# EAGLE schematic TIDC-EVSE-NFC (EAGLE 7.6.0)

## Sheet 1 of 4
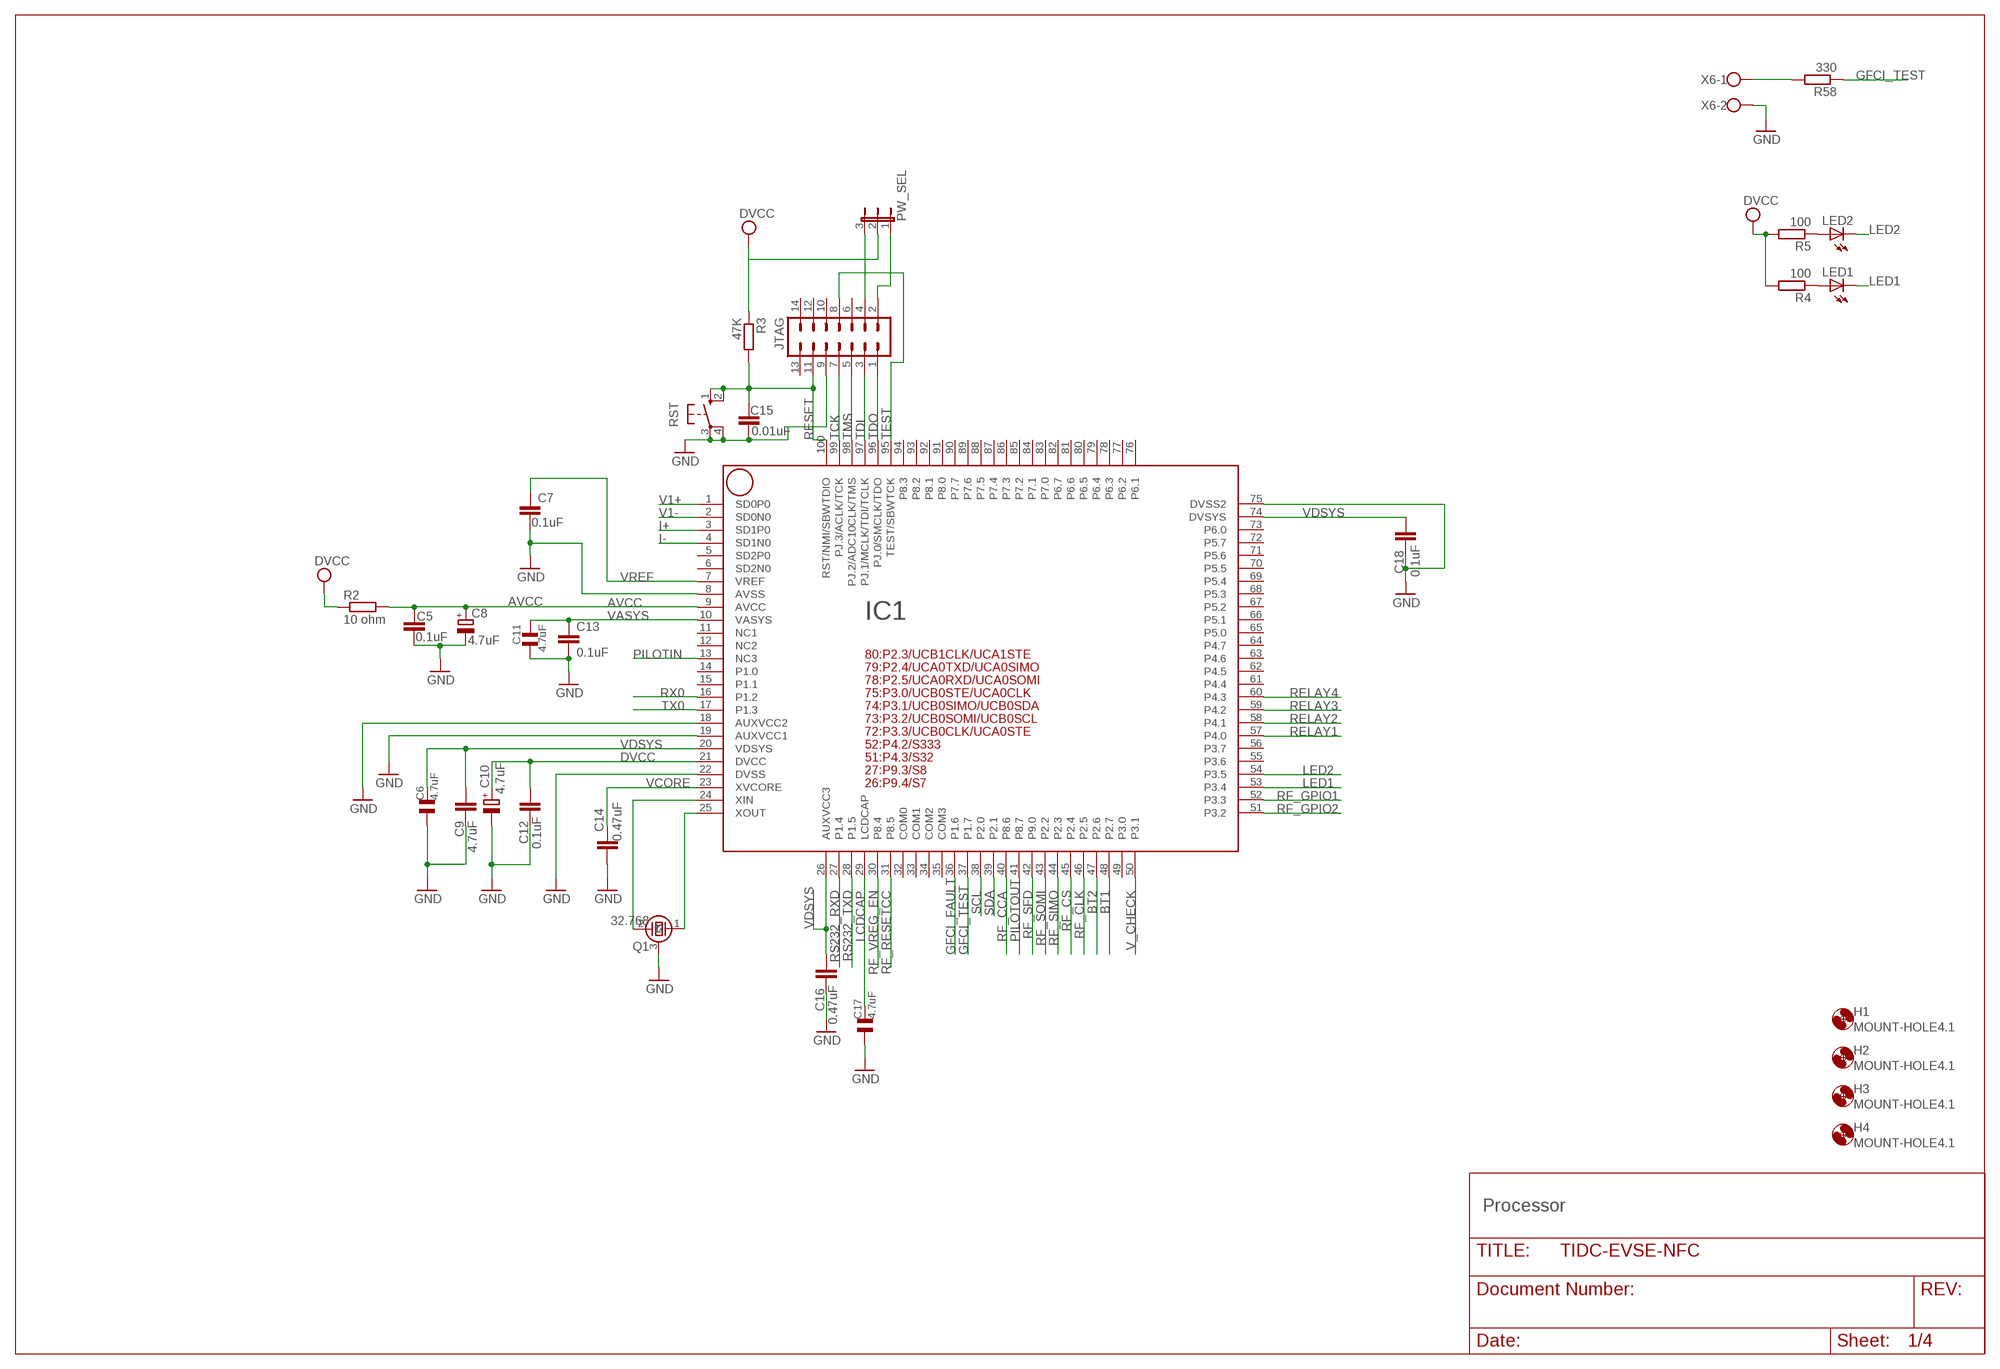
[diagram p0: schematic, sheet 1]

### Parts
C5  0.1uF  C-EUC0603  [C0603]
C6  4.7uF  C_0805  [0805]
C7  0.1uF  C-EUC0603  [C0603]
C8  4.7uF  CPOL-EUSMCB  [SMC_B]
C9  4.7uF  C-EUC0603  [C0603]
C10  4.7uF  CPOL-EUSMCB  [SMC_B]
C11  4.7uF  C_0805  [0805]
C12  0.1uF  C-EUC0603  [C0603]
C13  0.1uF  C-EUC0603  [C0603]
C14  0.47uF  C-EUC0603  [C0603]
C15  0.01uF  C-EUC0603  [C0603]
C16  0.47uF  C-EUC0603  [C0603]
C17  4.7uF  C_0805  [0805]
C18  0.1uF  C-EUC0603  [C0603]
H1  MOUNT-HOLE4.1  [4,1]
H2  MOUNT-HOLE4.1  [4,1]
H3  MOUNT-HOLE4.1  [4,1]
H4  MOUNT-HOLE4.1  [4,1]
IC1  F6733---PZ100  [PZ100]
JTAG  MA07-2MA07-2JTAG  [MA07-2JTAG]
LED1  LED3MM  [LED3MM]
LED2  LED3MM  [LED3MM]
PW_SEL  JP2E  [JP2]
Q1  32.768  CRYSTAL-LSDTC26H-1  [TC26H-1]
R2  10 ohm  R-EU_R0603  [R0603]
R3  47K  R-EU_R0603  [R0603]
R4  100  R-EU_R0603  [R0603]
R5  100  R-EU_R0603  [R0603]
R58  330  R-EU_R0603  [R0603]
RST  10-XX  [B3F-10XX]
X6  W237-102  [W237-102]

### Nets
AVCC: C5.1 C8.+ IC1.9(AVCC) R2.2 ; also sheet 4
BT1: IC1.48(P2.7) ; also sheet 2
BT2: IC1.47(P2.6) ; also sheet 2
DVCC: C10.+ C12.2 IC1.21(DVCC) PW_SEL.2 R2.1 R3.1 R4.2 R5.2 ; also sheet 2,3,4
GFCI_FAULT: IC1.36(P1.6) ; also sheet 4
GFCI_TEST: IC1.37(P1.7) R58.1
GND: C5.2 C6.1 C7.2 C8.- C9.1 C10.- C11.1 C12.1 C13.2 C14.1 C15.2 C16.1 C17.1 C18.1 IC1.8(AVSS) IC1.18(AUXVCC2) IC1.19(AUXVCC1) IC1.22(DVSS) IC1.75(DVSS2) JTAG.9 Q1.3 RST.3(P) RST.4(P1) X6.2 ; also sheet 2,3,4
I+: IC1.3(SD1P0) ; also sheet 4
I-: IC1.4(SD1N0) ; also sheet 4
JTAG_EXT: JTAG.4 PW_SEL.3
JTAG_INT: JTAG.2 PW_SEL.1
LCDCAP: C17.2 IC1.29(LCDCAP)
LED1: IC1.53(P3.4) LED1.K(C)
LED2: IC1.54(P3.5) LED2.K(C)
N$6: R58.2 X6.1
N$104: LED1.A R4.1
N$105: LED2.A R5.1
PILOTIN: IC1.13(NC3) ; also sheet 2
PILOTOUT: IC1.41(P8.7) ; also sheet 2
RELAY1: IC1.57(P4.0) ; also sheet 4
RELAY2: IC1.58(P4.1) ; also sheet 4
RELAY3: IC1.59(P4.2) ; also sheet 4
RELAY4: IC1.60(P4.3) ; also sheet 4
RESET: C15.1 IC1.100(RST/NMI/SBWTDIO) JTAG.11 R3.2 RST.1(S) RST.2(S1)
RF_CCA: IC1.40(P8.6) ; also sheet 2
RF_CLK: IC1.46(P2.5) ; also sheet 2
RF_CS: IC1.45(P2.4) ; also sheet 2
RF_GPIO1: IC1.52(P3.3) ; also sheet 2
RF_GPIO2: IC1.51(P3.2) ; also sheet 2
RF_RESETCC: IC1.31(P8.5) ; also sheet 2
RF_SFD: IC1.42(P9.0) ; also sheet 2
RF_SIMO: IC1.44(P2.3) ; also sheet 2
RF_SOMI: IC1.43(P2.2) ; also sheet 2
RF_VREG_EN: IC1.30(P8.4) ; also sheet 2
RS232_RXD: IC1.27(P1.4)
RS232_TXD: IC1.28(P1.5)
RX0: IC1.16(P1.2) ; also sheet 2
SCL: IC1.38(P2.0) ; also sheet 2
SDA: IC1.39(P2.1) ; also sheet 2
TCK: IC1.99(PJ.3/ACLK/TCK) JTAG.7
TDI: IC1.97(PJ.1/MCLK/TDI/TCLK) JTAG.3
TDO: IC1.96(PJ.0/SMCLK/TDO) JTAG.1
TEST: IC1.95(TEST/SBWTCK) JTAG.8
TMS: IC1.98(PJ.2/ADC10CLK/TMS) JTAG.5
TX0: IC1.17(P1.3) ; also sheet 2
V1+: IC1.1(SD0P0) ; also sheet 4
V1-: IC1.2(SD0N0) ; also sheet 4
V_CHECK: IC1.50(P3.1) ; also sheet 4
VASYS: C11.2 C13.1 IC1.10(VASYS)
VCORE: C14.2 IC1.23(XVCORE)
VDSYS: C6.2 C9.2 C16.2 C18.2 IC1.20(VDSYS) IC1.26(AUXVCC3) IC1.74(DVSYS)
VREF: C7.1 IC1.7(VREF)
XIN1: IC1.24(XIN) Q1.2
XOUT1: IC1.25(XOUT) Q1.1
Unconnected: IC1.5(SD2P0) IC1.6(SD2N0) IC1.11(NC1) IC1.12(NC2) IC1.14(P1.0) IC1.15(P1.1) IC1.32(COM0) IC1.33(COM1) IC1.34(COM2) IC1.35(COM3) IC1.49(P3.0) IC1.55(P3.6) IC1.56(P3.7) IC1.61(P4.4) IC1.62(P4.5) IC1.63(P4.6) IC1.65(P5.0) IC1.66(P5.1) IC1.68(P5.3) IC1.69(P5.4) IC1.70(P5.5) IC1.71(P5.6) IC1.72(P5.7) IC1.73(P6.0) IC1.76(P6.1) IC1.77(P6.2) IC1.78(P6.3) IC1.79(P6.4) IC1.80(P6.5) IC1.81(P6.6) IC1.82(P6.7) IC1.83(P7.0) IC1.84(P7.1) IC1.85(P7.2) IC1.86(P7.3) IC1.87(P7.4) IC1.88(P7.5) IC1.89(P7.6) IC1.90(P7.7) IC1.91(P8.0) IC1.93(P8.2) IC1.94(P8.3) JTAG.6 JTAG.10 JTAG.12 JTAG.13 JTAG.14

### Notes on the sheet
- Processor

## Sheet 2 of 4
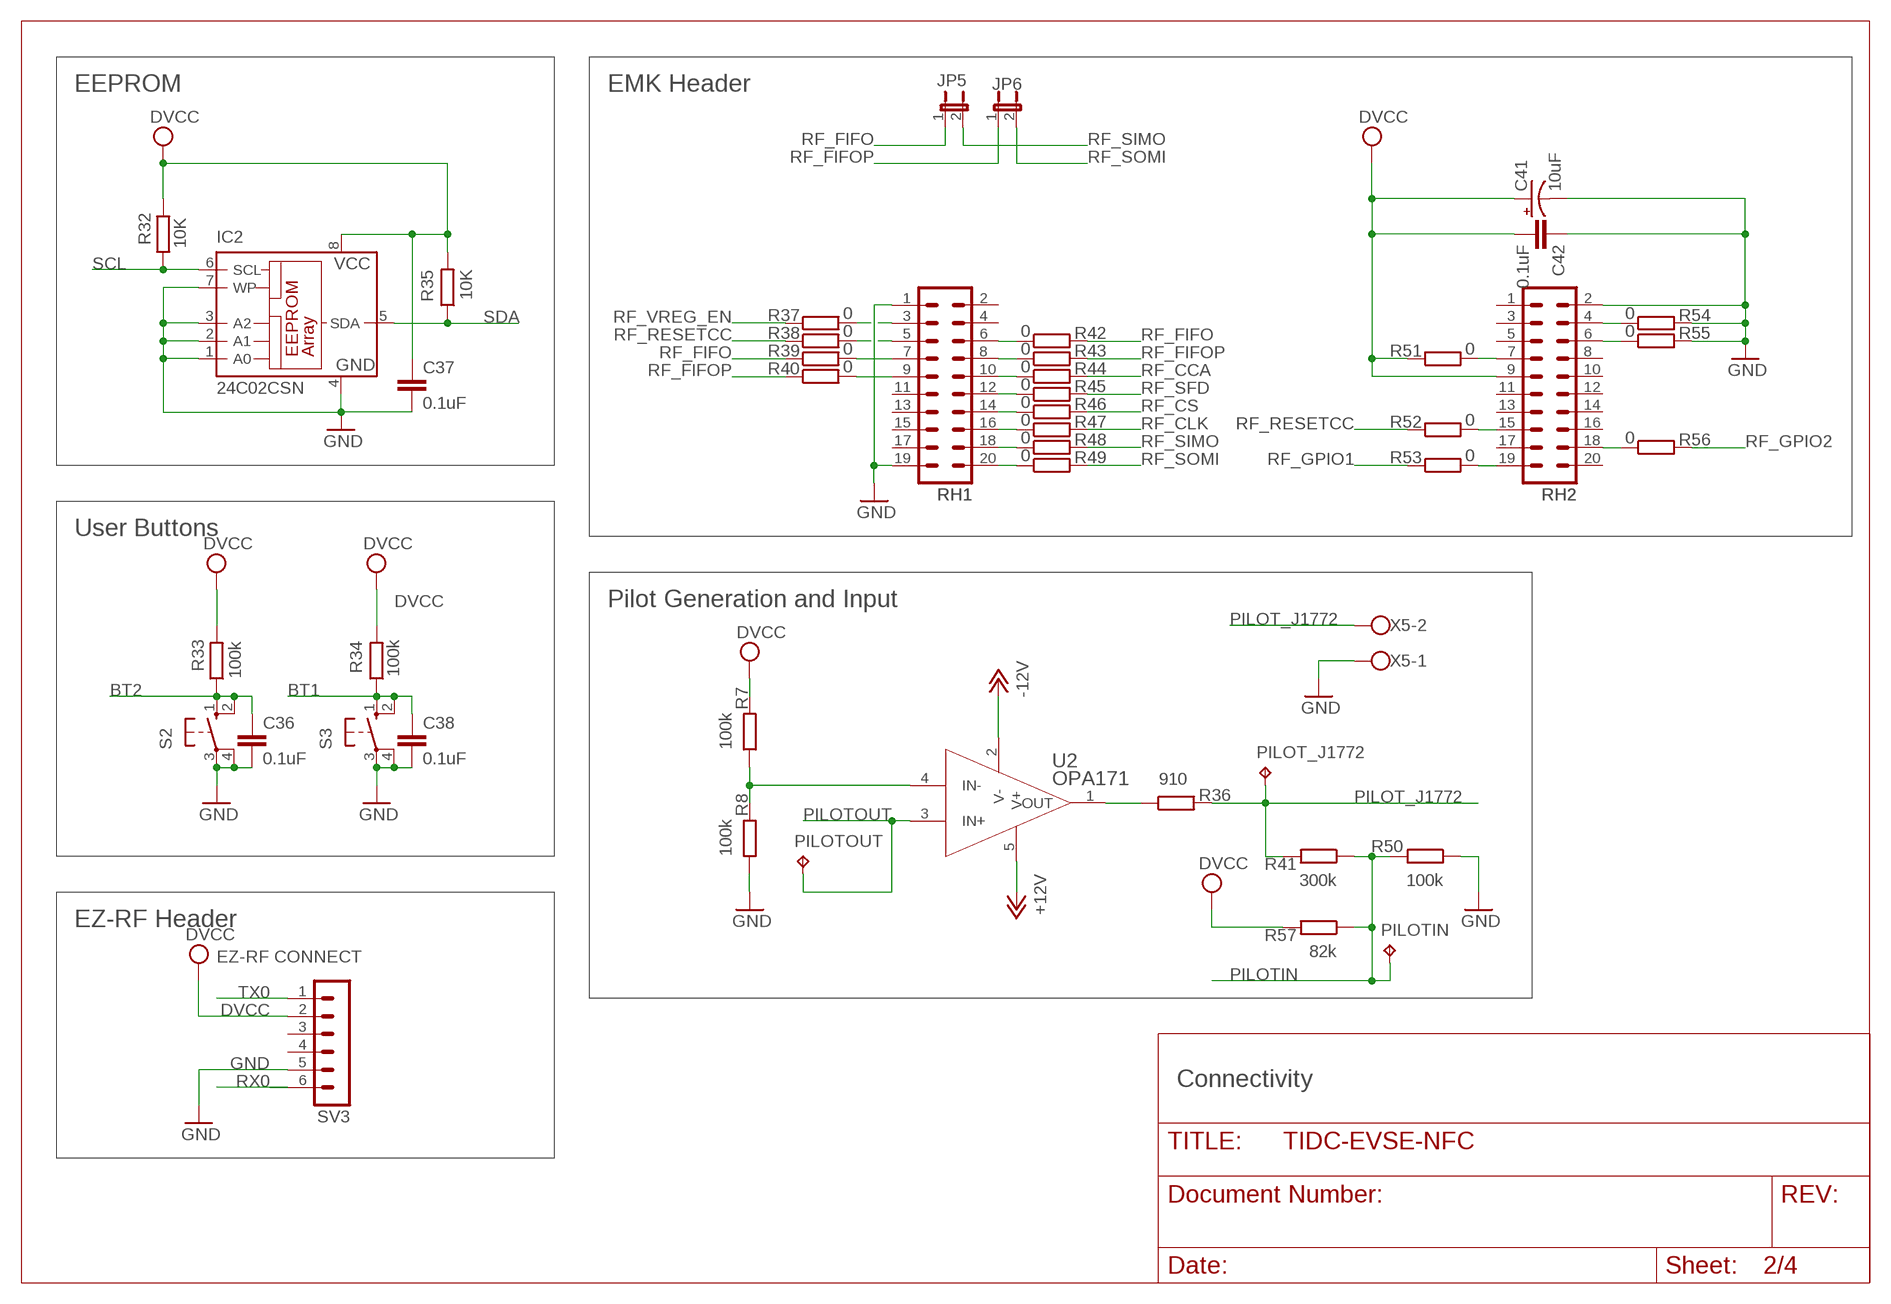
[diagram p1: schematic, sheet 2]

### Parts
C36  0.1uF  C-EUC0603  [C0603]
C37  0.1uF  C-EUC0603  [C0603]
C38  0.1uF  C-EUC0603  [C0603]
C41  10uF  CPOL-USCT3216  [CT3216]
C42  0.1uF  C-EUC0603  [C0603]
IC2  24C02CSN  [SO-08]
JP5  JP1E  [JP1]
JP6  JP1E  [JP1]
PILOT_J1772  TPB1,27  [B1,27]
PILOTIN  TPB1,27  [B1,27]
PILOTOUT  TPB1,27  [B1,27]
R7  100k  R-EU_R0603  [R0603]
R8  100k  R-EU_R0603  [R0603]
R32  10K  R-EU_R0603  [R0603]
R33  100k  R-EU_R0603  [R0603]
R34  100k  R-EU_R0603  [R0603]
R35  10K  R-EU_R0603  [R0603]
R36  910  R-EU_R0603  [R0603]
R37  0  R-EU_R0603  [R0603]
R38  0  R-EU_R0603  [R0603]
R39  0  R-EU_R0603  [R0603]
R40  0  R-EU_R0603  [R0603]
R41  300k  R-EU_R0603  [R0603]
R42  0  R-EU_R0603  [R0603]
R43  0  R-EU_R0603  [R0603]
R44  0  R-EU_R0603  [R0603]
R45  0  R-EU_R0603  [R0603]
R46  0  R-EU_R0603  [R0603]
R47  0  R-EU_R0603  [R0603]
R48  0  R-EU_R0603  [R0603]
R49  0  R-EU_R0603  [R0603]
R50  100k  R-EU_R0603  [R0603]
R51  0  R-EU_R0603  [R0603]
R52  0  R-EU_R0603  [R0603]
R53  0  R-EU_R0603  [R0603]
R54  0  R-EU_R0603  [R0603]
R55  0  R-EU_R0603  [R0603]
R56  0  R-EU_R0603  [R0603]
R57  82k  R-EU_R0603  [R0603]
RH1  TFM-110-02-SM-D-A-K  [TFM-110-02-SM-D-A-K]
RH2  TFM-110-02-SM-D-A-K  [TFM-110-02-SM-D-A-K]
S2  10-XX  [B3F-10XX]
S3  10-XX  [B3F-10XX]
SV3  MA06-1MA06-1-1.27  [MA06-1-1.27]
U2  OPA171  OPA171_DBV_5  [DBV5]
X5  W237-102  [W237-102]

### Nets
+12V: U2.5(V+) ; also sheet 3,4
-12V: U2.2(V-) ; also sheet 3
BT1: C38.1 R34.1 S3.1(S) S3.2(S1) ; also sheet 1
BT2: C36.1 R33.1 S2.1(S) S2.2(S1) ; also sheet 1
DVCC: C37.1 C41.+ C42.2 IC2.8(VCC) R7.2 R32.2 R33.2 R34.2 R35.2 R51.1 R57.2 RH2.9 SV3.2 ; also sheet 1,3,4
GND: C36.2 C37.2 C38.2 C41.- C42.1 IC2.1(A0) IC2.2(A1) IC2.3(A2) IC2.4(GND) IC2.7(WP) R8.1 R50.1 R54.2 R55.2 RH1.1 RH1.19 RH2.2 S2.3(P) S2.4(P1) S3.3(P) S3.4(P1) SV3.5 X5.1 ; also sheet 1,3,4
N$2: R7.1 R8.2 U2.4(IN-)
N$4: R36.1 U2.1(OUT)
N$35: R37.2 RH1.3
N$45: R38.2 RH1.5
N$50: R51.2 RH2.7
N$51: R54.1 RH2.4
N$52: R52.2 RH2.15
N$53: R55.1 RH2.6
N$55: R44.1 RH1.10
N$56: R45.1 RH1.12
N$57: R46.1 RH1.14
N$59: R47.1 RH1.16
N$60: R48.1 RH1.18
N$61: R49.1 RH1.20
N$81: R53.2 RH2.19
N$83: R56.1 RH2.18
N$85: R39.2 RH1.7
N$86: R40.2 RH1.9
N$87: R43.1 RH1.8
N$88: R42.1 RH1.6
PILOT_J1772: PILOT_J1772.TP R36.2 R41.2 X5.2
PILOTIN: PILOTIN.TP R41.1 R50.2 R57.1 ; also sheet 1
PILOTOUT: PILOTOUT.TP U2.3(IN+) ; also sheet 1
RF_CCA: R44.2 ; also sheet 1
RF_CLK: R47.2 ; also sheet 1
RF_CS: R46.2 ; also sheet 1
RF_FIFO: JP5.1 R39.1 R42.2
RF_FIFOP: JP6.1 R40.1 R43.2
RF_GPIO1: R53.1 ; also sheet 1
RF_GPIO2: R56.2 ; also sheet 1
RF_RESETCC: R38.1 R52.1 ; also sheet 1
RF_SFD: R45.2 ; also sheet 1
RF_SIMO: JP5.2 R48.2 ; also sheet 1
RF_SOMI: JP6.2 R49.2 ; also sheet 1
RF_VREG_EN: R37.1 ; also sheet 1
RX0: SV3.6 ; also sheet 1
SCL: IC2.6(SCL) R32.1 ; also sheet 1
SDA: IC2.5(SDA) R35.1 ; also sheet 1
TX0: SV3.1 ; also sheet 1
Unconnected: RH1.2 RH1.4 RH1.11 RH1.13 RH1.15 RH1.17 RH2.1 RH2.3 RH2.5 RH2.8 RH2.10 RH2.11 RH2.12 RH2.13 RH2.14 RH2.16 RH2.17 RH2.20 SV3.3 SV3.4

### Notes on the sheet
- EEPROM | EMK Header
- User Buttons
- Pilot Generation and Input
- EZ-RF Header
- EZ-RF CONNECT
- Connectivity

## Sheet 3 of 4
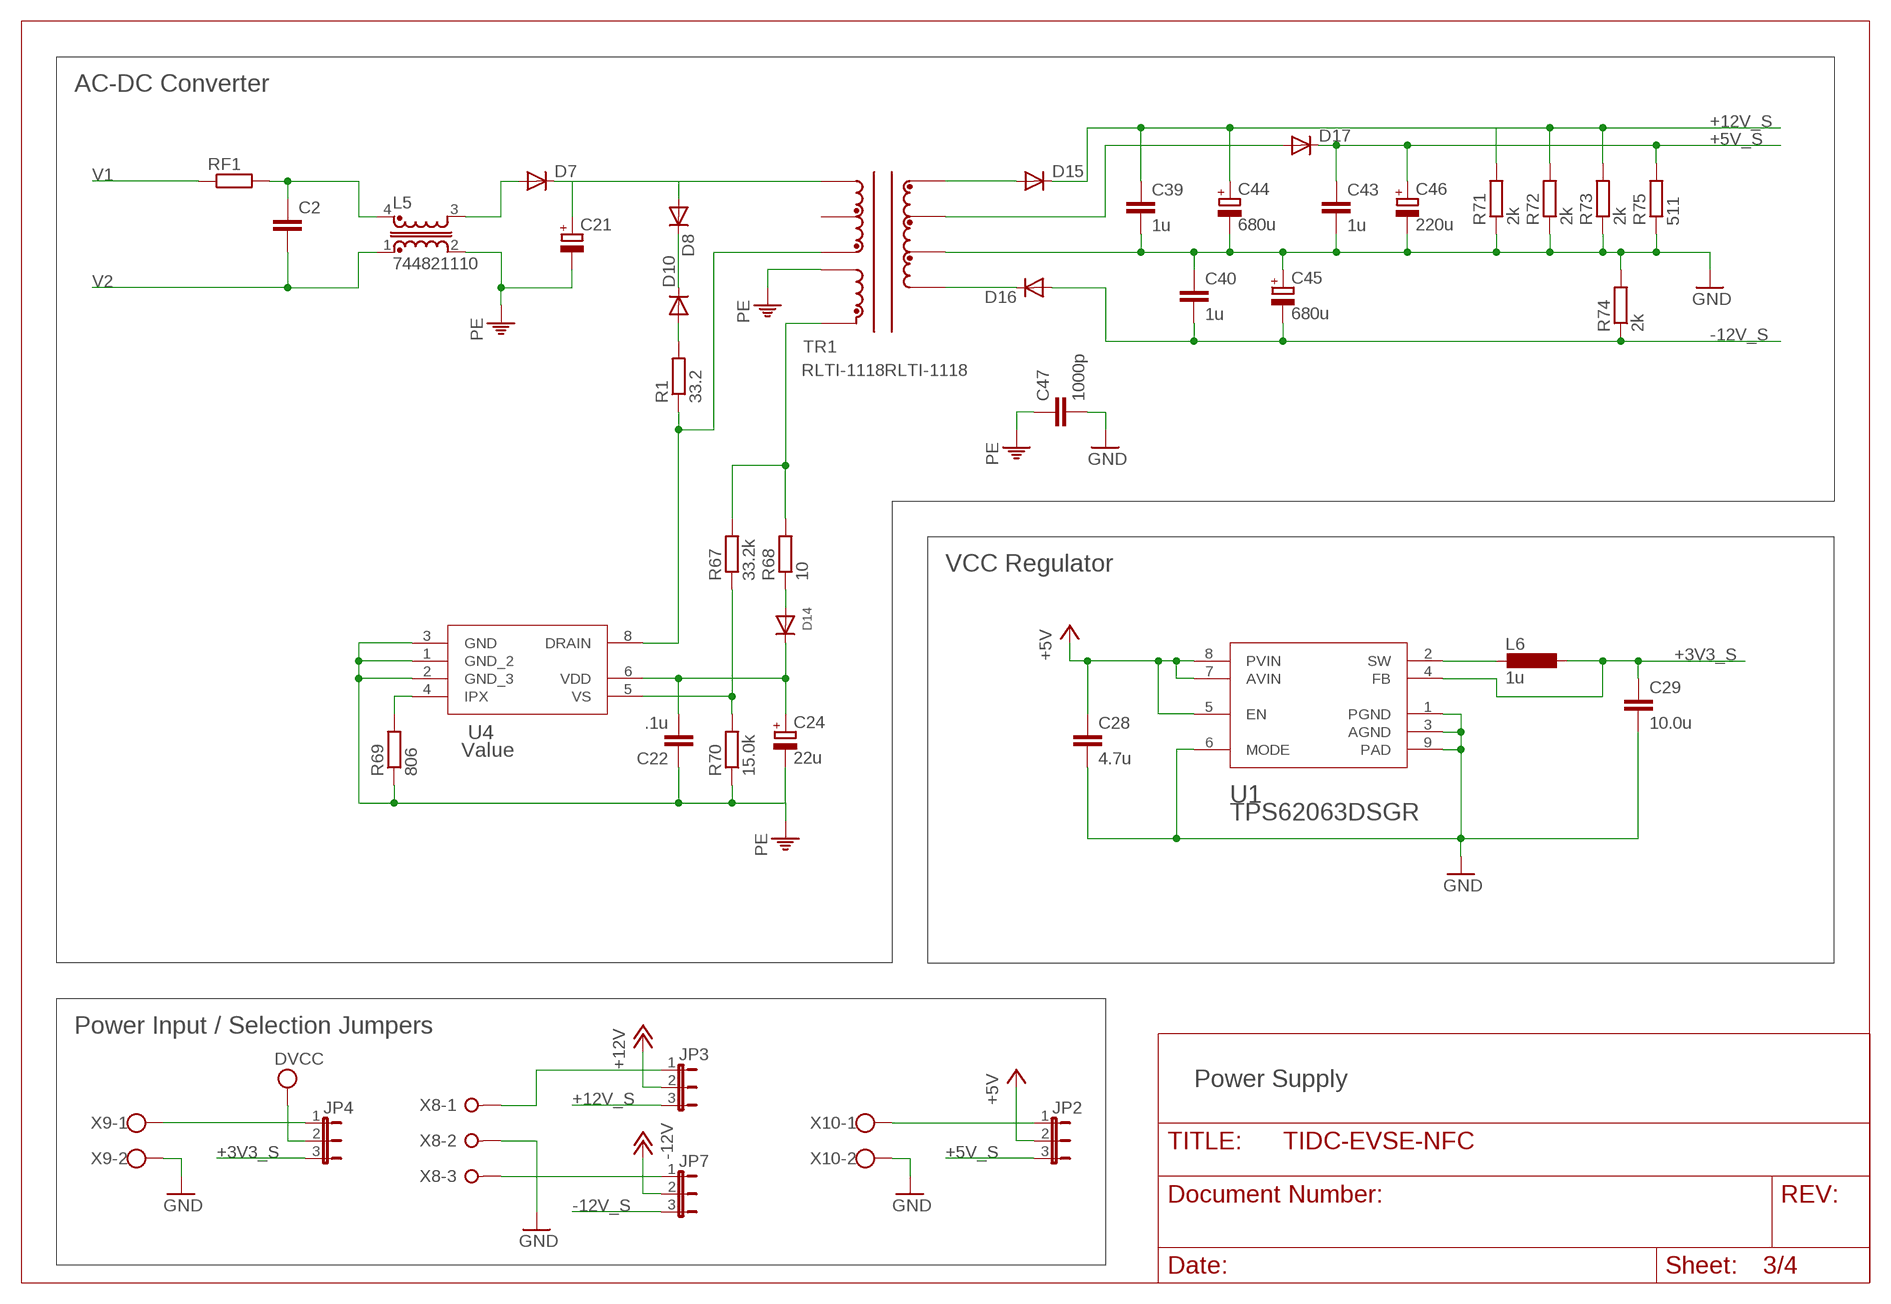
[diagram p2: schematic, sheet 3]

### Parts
C2  C-EU102-064X133  [C102-064X133]
C21  CPOL-EUE7.5-16  [E7,5-16]
C22  .1u  C-EUC0603  [C0603]
C24  22u  CPOL-EUE2.5-5  [E2,5-5]
C28  4.7u  C-EUC0805  [C0805]
C29  10.0u  C-EUC0603  [C0603]
C39  1u  C-EUC0805  [C0805]
C40  1u  C-EUC0805  [C0805]
C43  1u  C-EUC0805  [C0805]
C44  680u  CPOL-EUE5-10.5  [E5-10,5]
C45  680u  CPOL-EUE5-10.5  [E5-10,5]
C46  220u  CPOL-EUE2.5-6  [E2,5-6]
C47  1000p  C-EU075-032X103  [C075-032X103]
D7  DIODE-DO214AC  [DO214AC]
D8  DIODE-DO214AA  [DO214AA]
D10  DIODE-DO214AC  [DO214AC]
D14  DIODESOD-323F  [SOD-323F]
D15  DIODE-DO214AA  [DO214AA]
D16  DIODE-DO214AA  [DO214AA]
D17  DIODE-DO-214AC  [DO-214AC]
JP2  JP2E  [JP2]
JP3  JP2E  [JP2]
JP4  JP2E  [JP2]
JP7  JP2E  [JP2]
L5  744821110  [744821110]
L6  1u  SRN3015  [SRN3015]
R1  33.2  R-EU_R0805  [R0805]
R67  33.2k  R-EU_R0603  [R0603]
R68  10  R-EU_R0603  [R0603]
R69  806  R-EU_R0603  [R0603]
R70  15.0k  R-EU_R0603  [R0603]
R71  2k  R-EU_R0805  [R0805]
R72  2k  R-EU_R0805  [R0805]
R73  2k  R-EU_R0805  [R0805]
R74  2k  R-EU_R0805  [R0805]
R75  511  R-EU_R0805  [R0805]
RF1  R-EU_0411/12  [0411/12]
TR1  RLTI-1118RLTI-1118  [RLTI-1118]
U1  TPS62063DSGR  [DSG0008A]
U4  Value  UCC28910D  [D0007A]
X8  W237-03P  [W237-133]
X9  W237-102  [W237-102]
X10  W237-102  [W237-102]

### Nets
+3V3_S: C29.1 JP4.3 L6.V_1 U1.4(FB)
+5V: C28.1 JP2.2 U1.5(EN) U1.7(AVIN) U1.8(PVIN)
+5V_S: C43.1 C46.+ D17.C JP2.3 R75.2
+12V: JP3.2 ; also sheet 2,4
+12V_S: C39.1 C44.+ D15.C JP3.3 R71.2 R72.2 R73.2
-12V: JP7.2 ; also sheet 2
-12V_S: C40.2 C45.- D16.A JP7.3 R74.1
DVCC: JP4.2 ; also sheet 1,2,4
GND: C28.2 C29.2 C39.2 C40.1 C43.2 C44.- C45.+ C46.- C47.2 R71.1 R72.1 R73.1 R74.2 R75.1 TR1.V_7 U1.1(PGND) U1.3(AGND) U1.6(MODE) U1.9(PAD) X8.2 X9.2 X10.2 ; also sheet 1,2,4
N$1: L6.V_2 U1.2(SW)
N$3: JP3.1 X8.1
N$7: JP7.1 X8.3
N$12: JP4.1 X9.1
N$13: JP2.1 X10.1
N$15: C2.1 L5.4 RF1.2
N$18: D7.A L5.3
N$20: C21.+ D7.C D8.A TR1.V_1
N$22: D8.C D10.C
N$24: D10.A R1.2
N$30: R1.1 TR1.V_3 U4.8(DRAIN)
N$36: R67.2 R68.2 TR1.V_5
N$37: D14.A R68.1
N$38: C22.2 C24.+ D14.C U4.6(VDD)
N$40: D16.C TR1.V_6
N$41: D15.A TR1.V_10
N$43: D17.A TR1.V_8
N$48: R67.1 R70.2 U4.5(VS)
N$49: R69.2 U4.4(IPX)
PE: C21.- C22.1 C24.- C47.1 L5.2 R69.1 R70.1 TR1.V_4 U4.1(GND_2) U4.2(GND_3) U4.3(GND)
V1: RF1.1 ; also sheet 4
V2: C2.2 L5.1 ; also sheet 4
Unconnected: TR1.V_2

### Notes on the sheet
- AC-DC Converter
- VCC Regulator
- Power Input / Selection Jumpers
- Power Supply

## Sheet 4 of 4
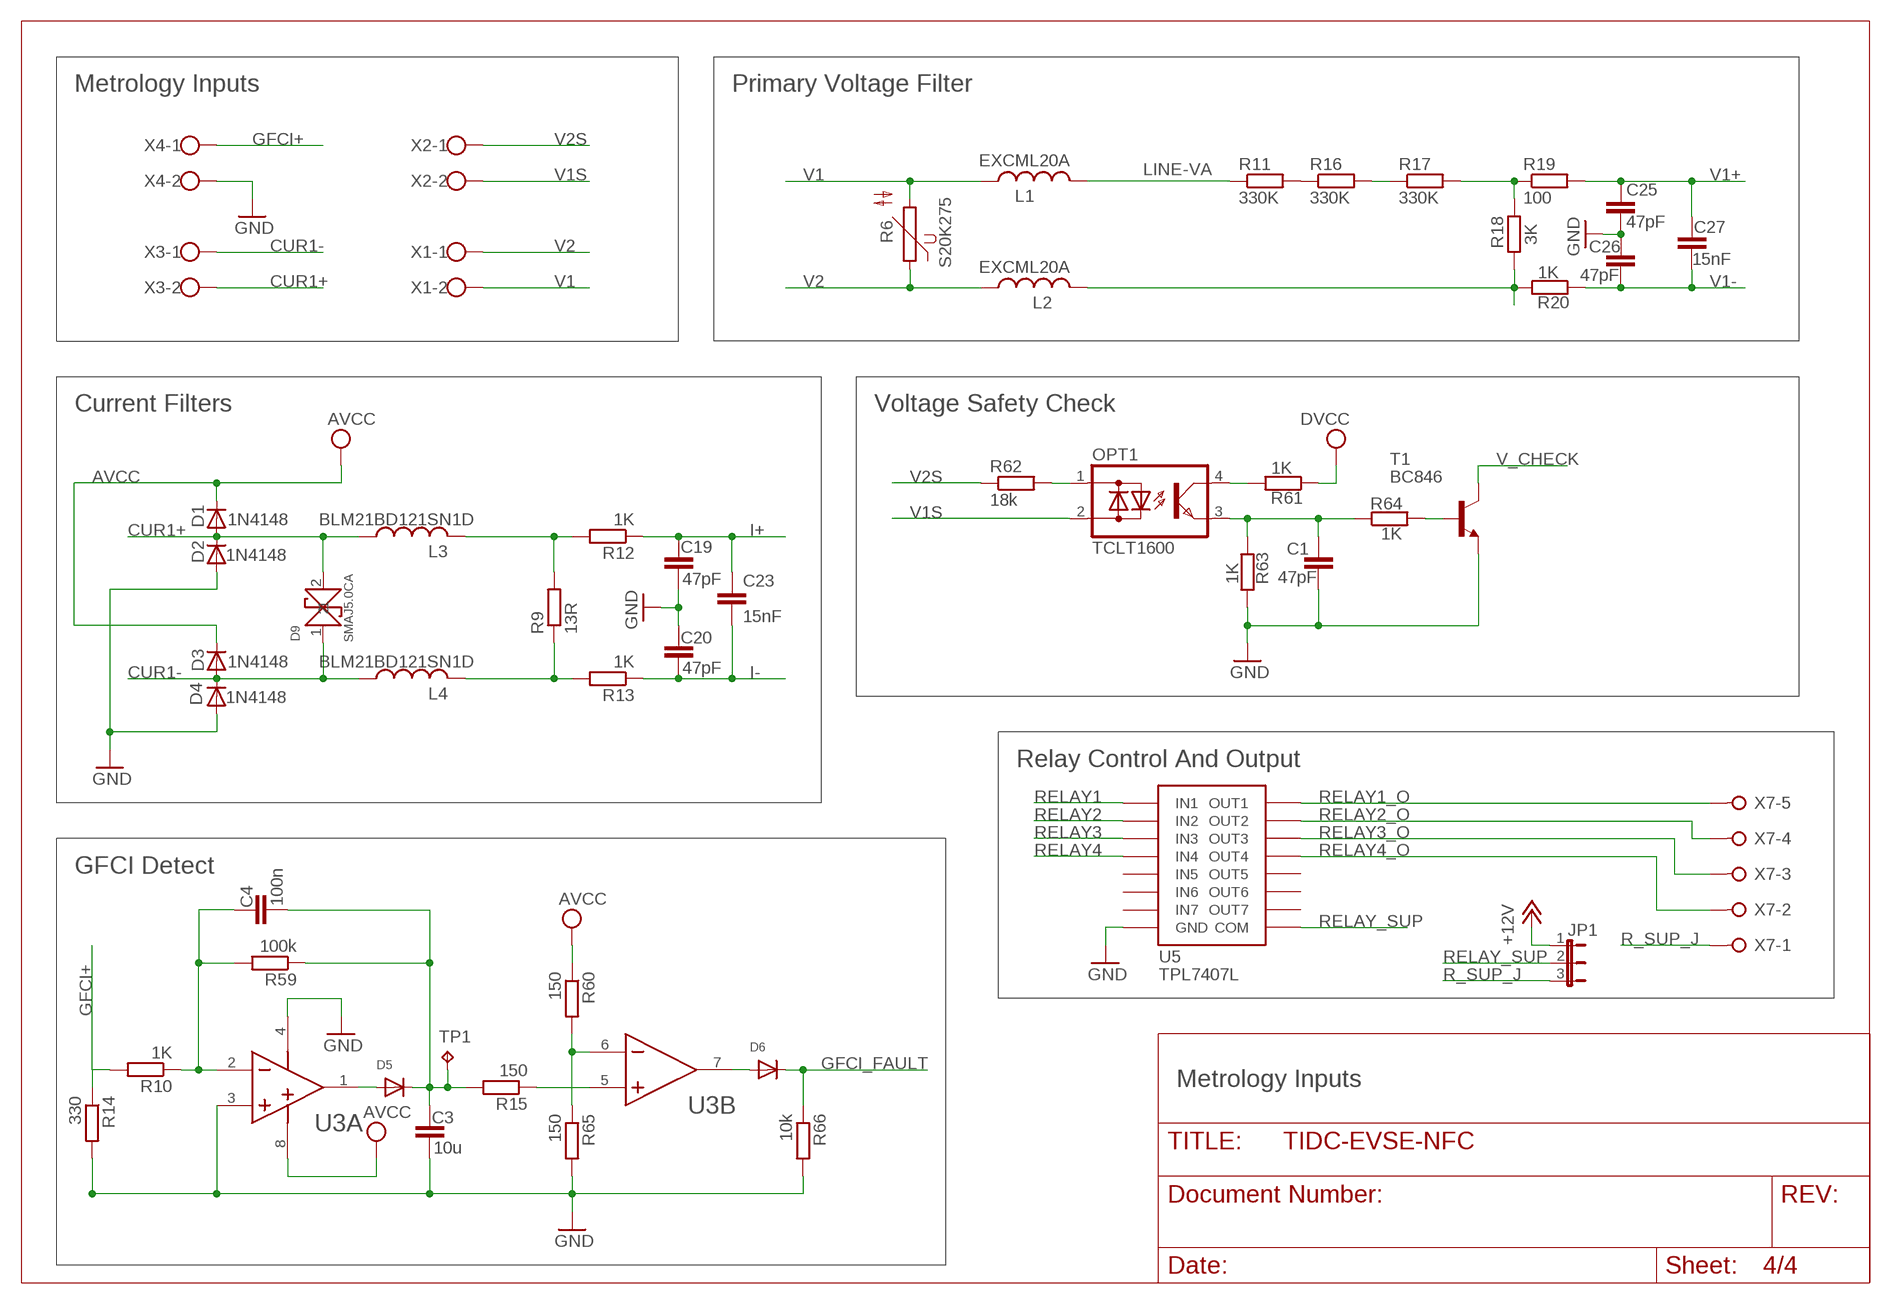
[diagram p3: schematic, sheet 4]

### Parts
C1  47pF  C-EUC0603  [C0603]
C3  10u  C-EUC0603  [C0603]
C4  100n  C-EUC0603  [C0603]
C19  47pF  C-EUC0603  [C0603]
C20  47pF  C-EUC0603  [C0603]
C23  15nF  C-EUC0603  [C0603]
C25  47pF  C-EUC0603  [C0603]
C26  47pF  C-EUC0603  [C0603]
C27  15nF  C-EUC0603  [C0603]
D1  1N4148  1N4148SOD80C  [SOD80C]
D2  1N4148  1N4148SOD80C  [SOD80C]
D3  1N4148  1N4148SOD80C  [SOD80C]
D4  1N4148  1N4148SOD80C  [SOD80C]
D5  DIODESOD-123  [SOD-123]
D6  DIODESOD-123  [SOD-123]
D9  SMAJ5.0CA  SMAJ  [DO-214]
JP1  JP2E  [JP2]
L1  EXCML20A  L-US08050805  [0805@1]
L2  EXCML20A  L-US08050805  [0805@1]
L3  BLM21BD121SN1D  L-USL2012C  [L2012C]
L4  BLM21BD121SN1D  L-USL2012C  [L2012C]
OPT1  TCLT1600  [TCLT1600]
R6  S20K275  S20K680S20K680-1  [S20K680-1]
R9  13R  R-EU_R0603  [R0603]
R10  1K  R-EU_R0603  [R0603]
R11  330K  R-EU_R0603  [R0603]
R12  1K  R-EU_R0603  [R0603]
R13  1K  R-EU_R0603  [R0603]
R14  330  R-EU_R0603  [R0603]
R15  150  R-EU_R0603  [R0603]
R16  330K  R-EU_R0603  [R0603]
R17  330K  R-EU_R0603  [R0603]
R18  3K  R-EU_R0603  [R0603]
R19  100  R-EU_R0603  [R0603]
R20  1K  R-EU_R0603  [R0603]
R59  100k  R-EU_R0603  [R0603]
R60  150  R-EU_R0603  [R0603]
R61  1K  R-EU_R0603  [R0603]
R62  18k  R-EU_R2512  [R2512]
R63  1K  R-EU_R0603  [R0603]
R64  1K  R-EU_R0603  [R0603]
R65  150  R-EU_R0603  [R0603]
R66  10k  R-EU_R0603  [R0603]
T1  BC846  [SOT23]
TP1  TPB1,27  [B1,27]
U3  LM7321  LM7321_DUAL  [M08A]
U5  TPL7407L  [TSSOP_16]
X1  W237-102  [W237-102]
X2  W237-102  [W237-102]
X3  W237-102  [W237-102]
X4  W237-102  [W237-102]
X7  W237-05P  [W237-5P]

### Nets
+12V: JP1.1 ; also sheet 2,3
AVCC: D1.C D3.C R60.1 U3.8(A:V+) ; also sheet 1
CUR1+: D1.A D2.C D9.2 L3.1 X3.2
CUR1-: D3.A D4.C D9.1 L4.1 X3.1
DVCC: R61.1 ; also sheet 1,2,3
GFCI+: R10.2 R14.1 X4.1
GFCI_FAULT: D6.C R66.1 ; also sheet 1
GND: C1.2 C3.2 C19.2 C20.1 C25.2 C26.1 D2.A D4.A R14.2 R63.2 R65.2 R66.2 T1.2(E) U3.3(A:IN1+) U3.4(A:V-) U5.V_8(GND) X4.2 ; also sheet 1,2,3
I+: C19.1 C23.1 R12.1 ; also sheet 1
I-: C20.2 C23.2 R13.1 ; also sheet 1
LINE-VA: L1.2 R11.1
N$5: C4.1 R10.1 R59.2 U3.2(A:IN1-)
N$8: D5.A U3.1(A:OUT1)
N$9: OPT1.1(AC1) R62.2
N$10: C1.1 OPT1.3(E) R63.1 R64.1
N$11: C3.1 C4.2 D5.C R15.2 R59.1 TP1.TP
N$14: OPT1.4(C) R61.2
N$16: R15.1 U3.5(B:IN2+)
N$17: R60.2 R65.1 U3.6(B:IN2-)
N$19: D6.A U3.7(B:OUT2)
N$21: R64.2 T1.1(B)
N$23: L2.2 R18.1 R20.2
N$25: R16.2 R17.1
N$27: L4.2 R9.1 R13.2
N$32: R17.2 R18.2 R19.1
N$39: R11.2 R16.1
N$42: L3.2 R9.2 R12.2
R_SUP_J: JP1.3 X7.1
RELAY1: U5.V_1(IN1) ; also sheet 1
RELAY1_O: U5.V_16(OUT1) X7.5
RELAY2: U5.V_2(IN2) ; also sheet 1
RELAY2_O: U5.V_15(OUT2) X7.4
RELAY3: U5.V_3(IN3) ; also sheet 1
RELAY3_O: U5.V_14(OUT3) X7.3
RELAY4: U5.V_4(IN4) ; also sheet 1
RELAY4_O: U5.V_13(OUT4) X7.2
RELAY_SUP: JP1.2 U5.V_9(COM)
V1: L1.1 R6.2 X1.2 ; also sheet 3
V1+: C25.1 C27.1 R19.2 ; also sheet 1
V1-: C26.2 C27.2 R20.1 ; also sheet 1
V1S: OPT1.2(AC2) X2.2
V2: L2.1 R6.1 X1.1 ; also sheet 3
V2S: R62.1 X2.1
V_CHECK: T1.3(C) ; also sheet 1
Unconnected: U5.V_5(IN5) U5.V_6(IN6) U5.V_7(IN7) U5.V_10(OUT7) U5.V_11(OUT6) U5.V_12(OUT5)

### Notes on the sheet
- Metrology Inputs | Primary Voltage Filter
- Current Filters | Voltage Safety Check
- Relay Control And Output
- GFCI Detect
- Metrology Inputs

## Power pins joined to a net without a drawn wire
P4.7: IC1.64(P4.7)
P5.2: IC1.67(P5.2)
P8.1: IC1.92(P8.1)

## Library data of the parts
C1 C3-C5 C7 C9 C12-C16 C18-C20 C23 C25-C27 C36-C38 = ElecMeter:C-EU: CAPACITOR, European symbol
C2 = rcl:C-EU: CAPACITOR, European symbol; DIGIKEY: 399-9643-ND
C6 C11 C17 = ssmd:C_0805
C8 C10 = ElecMeter:CPOL-EU: POLARIZED CAPACITOR, European symbol
C21 = rcl:CPOL-EU: POLARIZED CAPACITOR, European symbol; DIGIKEY: P5944-ND
C22 = ElecMeter:C-EU: CAPACITOR, European symbol; DIGIKEY: 478-5052-1-ND
C24 = rcl:CPOL-EU: POLARIZED CAPACITOR, European symbol; DIGIKEY: P15803CT-ND
C28 = rcl:C-EU: CAPACITOR, European symbol; DIGIKEY: 490-9750-1-ND
C29 = ElecMeter:C-EU: CAPACITOR, European symbol; DIGIKEY: 1276-1119-1-ND
C39 C40 C43 = rcl:C-EU: CAPACITOR, European symbol; DIGIKEY: 478-1409-1-ND
C41 = rcl:CPOL-US: POLARIZED CAPACITOR, American symbol
C42 = resistor:C-EU: CAPACITOR, European symbol
C44 C45 = rcl:CPOL-EU: POLARIZED CAPACITOR, European symbol; DIGIKEY: 1189-1255-ND
C46 = rcl:CPOL-EU: POLARIZED CAPACITOR, European symbol
C47 = rcl:C-EU: CAPACITOR, European symbol; MOUSER: 72-VY2102M29Y5UG63V7
D1-D4 = ElecMeter:1N4148: DIODE
D5 D6 = adafruit:DIODE: Diode; DIGIKEY: 1N4148WTPMSCT-ND
D7 = diode:DIODE-: DIODE; DIGIKEY: US1J-E3/5ATGICT-ND
D8 = diode:DIODE-: DIODE; DIGIKEY: 1SMB5952BT3GOSCT-ND
D9 = CON1:SMAJ
D10 = diode:DIODE-: DIODE; DIGIKEY: US1M-FDICT-ND
D14 = adafruit:DIODE: Diode; DIGIKEY: BAS20HT1GOSCT-ND
D15 D16 = diode:DIODE-: DIODE; DIGIKEY: B160B-FDICT-ND
D17 = diode:DIODE-: DIODE; DIGIKEY: B130L-FDICT-ND
H1-H4 = holes:MOUNT-HOLE: MOUNTING HOLE with drill center marker
IC1 = partslibTI_MSP430_v122:F6733---PZ100
IC2 = ElecMeter:24C*: Serial EEPROM 1 K/2 K/4 K
JP1-JP4 JP7 PW_SEL = custom_jumper:JP2E: JUMPER; DIGIKEY: 3M9322-ND
JP5 JP6 = custom_jumper:JP1E: JUMPER; DIGIKEY: 3M9447-ND
JTAG = ElecMeter:MA07-2: PIN HEADER; DIGIKEY: MHB14K-ND
L1 L2 = SMD:L-US0805
L3 L4 = ElecMeter:L-US: INDUCTOR, American symbol
L5 = 744821110Lbr:744821110; DIGIKEY: 732-1437-ND
L6 = BournsIndLbr:SRN3015
LED1 LED2 = ElecMeter:LED: LED; DIGIKEY: 511-1211-ND
OPT1 = TCLT1600:TCLT1600; DIGIKEY: TCLT1600CT-ND
PILOT_J1772 PILOTIN PILOTOUT TP1 = testpad:TP: Test pad
Q1 = ElecMeter:CRYSTAL-LSD
R1 = rcl:R-EU_: RESISTOR, European symbol; DIGIKEY: 541-33.2CCT-ND
R2-R5 R9-R20 R32-R35 R58-R61 R63-R66 = ElecMeter:R-EU_: RESISTOR, European symbol
R6 = ElecMeter:S20K680: VARISTOR
R7 R8 R37-R40 R42-R49 R51-R57 = rcl:R-EU_: RESISTOR, European symbol
R36 = rcl:R-EU_: RESISTOR, European symbol; DIGIKEY: P910GTR-ND
R41 = rcl:R-EU_: RESISTOR, European symbol; DIGIKEY: P300KDBCT-ND
R50 = rcl:R-EU_: RESISTOR, European symbol; DIGIKEY: P100KDBCT-ND
R62 = resistor:R-EU_: RESISTOR, European symbol; DIGIKEY: 7-2176070-9; SPICEPREFIX: R
R67 = rcl:R-EU_: RESISTOR, European symbol; DIGIKEY: 541-33.2KHCT-ND
R68 = rcl:R-EU_: RESISTOR, European symbol; DIGIKEY: 541-10.0HCT-ND
R69 = rcl:R-EU_: RESISTOR, European symbol; DIGIKEY: 541-806HCT-ND
R70 = rcl:R-EU_: RESISTOR, European symbol; DIGIKEY: 541-15.0KHCT-ND
R71-R74 = rcl:R-EU_: RESISTOR, European symbol; DIGIKEY: 541-2.0KTADKR-ND
R75 = rcl:R-EU_: RESISTOR, European symbol; DIGIKEY: YAG1923CT-ND
RF1 = rcl:R-EU_: RESISTOR, European symbol; DIGIKEY: 4.7DLCT-ND
RH1 RH2 = _MSP430:TFM-110-02-SM-D-A-K
RST S2 S3 = ElecMeter:10-XX: OMRON SWITCH
SV3 = con-lstb:MA06-1: PIN HEADER
T1 = transistor:BC846: NPN TRANSISTOR; DIGIKEY: BC846B-TPMSCT-ND
TR1 = RencoRLTI-1118:RLTI-1118
U1 = TPS62063lbr:TPS62063DSGR; COMPTYPE: IC; MANUFACTURER: Texas Instruments; MOUNTTYPE: SMT; PACKAGEREFERENCE: DSG0008A; PARTNUMBER: TPS62063DSG; PIN_COUNT: 9; ROHS: Y
U2 = OPA171Lib:OPA171_DBV_5; DATASHEETURL: http://www.ti.com/lit/gpn/OPA171; DESCRIPTION: 36V, Low Power, RRO, General Purpose Operational Amplifier in MicroPackages; FAMILY_NAME: RAIL-TO-RAIL; GENERIC_PART_NUMBER: OPA171; INDUSTRY_STD_PKG_TYPE: SOT-23; MANUFACTURER: Texas Instruments; MANUFACTURER_PART_NUMBER: opa171_dbv_5; PACKAGE_DESIGNATOR: DBV; PIN_COUNT: 5; VENDOR: Texas Instruments
U3 = LM7321Lbr:LM7321_DUAL; DIGIKEY: LM7321MAX/NOPBCT-ND
U4 = UCC28910 Lbr:UCC28910D; COMPTYPE: IC; MANUFACTURER: Texas Instruments; MOUNTTYPE: SMT; PACKAGEREFERENCE: D0007A; PARTNUMBER: UCC28910D; PIN_COUNT: 7; REFDES: RefDes; ROHS: Y; TYPE: TYPE
U5 = tpl7407lLbr:TPL7407L; DIGIKEY: 296-37285-1-ND
X1-X6 X9 X10 = con-wago-500:W237-102: WAGO SCREW CLAMP; MPN: 237-102; OC_FARNELL: unknown; OC_NEWARK: 70K9898
X7 = con-wago-508:W237-05P: WAGO SREW CLAMP; OC_FARNELL: unknown; OC_NEWARK: unknown
X8 = con-wago-508:W237-03P: WAGO SREW CLAMP; OC_FARNELL: unknown; OC_NEWARK: unknown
